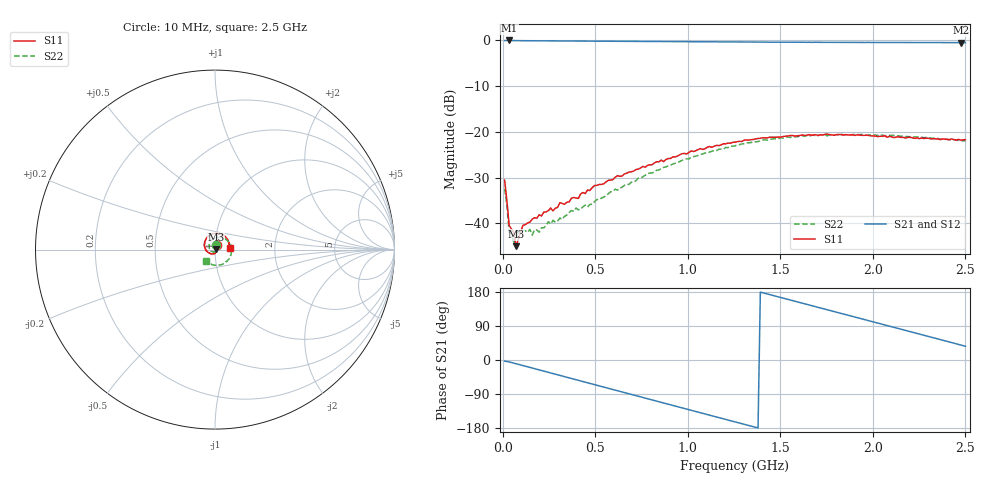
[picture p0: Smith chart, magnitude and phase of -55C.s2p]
!Agilent Technologies,E8364B,MY43040864,A.07.50.48
!Agilent E8364B: A.07.50.48
!Date: Tuesday, September 09, 2025 17:34:12
!Correction: S11(Full 2 Port(1,2))
!S21(Full 2 Port(1,2))
!S12(Full 2 Port(1,2))
!S22(Full 2 Port(1,2))
!S2P File: Measurements: S11, S21, S12, S22:
# Hz S  dB  R 50
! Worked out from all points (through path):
!   201 points, 10 MHz to 2.5 GHz, reference 50 ohm
!   highest |S21| = -0.01 dB at 34.9 MHz (marker M1); lowest = -0.5 dB at 2.475 GHz (marker M2)
!   group delay of S21, straight-line fit = 359 ps
!   lowest |S11| = -45.0 dB at 72.25 MHz (marker M3), VSWR 1.01, Z = 50.6 + j0.134 ohm
!   |S11| at or under -10 dB: start of sweep to end of sweep
!   |S22| runs from -44.5 to -20.5 dB; largest |S21 - S12| = 0.0037
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1e7  -30.53 68.7  -0.03 -2.9  -0.03 -2.9  -32.42 79.3
2.245e7  -35.14 59.1  -0.03 -4.0  -0.04 -4.0  -36.00 70.6
3.49e7  -40.49 52.3  -0.01 -5.2  -0.02 -5.1  -42.06 55.7
4.735e7  -41.23 46.1  -0.03 -6.7  -0.05 -6.7  -42.39 26.8
5.98e7  -42.03 29.8  -0.04 -8.3  -0.07 -8.4  -44.47 37.0
7.225e7  -44.98 13.6  -0.06 -9.9  -0.06 -9.9  -41.28 21.1
1.096e8  -40.39 10.1  -0.07 -14.9  -0.07 -14.8  -41.46 17.6
1.4695e8  -39.70 -18.3  -0.07 -19.6  -0.10 -19.6  -41.30 -20.6
1.594e8  -39.06 -26.3  -0.09 -21.3  -0.09 -21.2  -42.56 -22.2
2.4655e8  -37.21 -54.2  -0.11 -32.6  -0.11 -32.6  -39.62 -57.1
4.333e8  -33.25 -99.3  -0.15 -56.9  -0.16 -56.8  -36.36 -112.4
6.325e8  -29.73 -136.2  -0.20 -82.7  -0.21 -82.8  -32.32 -167.0
8.4415e8  -26.54 -169.7  -0.25 -110.1  -0.25 -110.2  -28.32 147.2
1.06825e9  -23.65 155.7  -0.30 -139.2  -0.30 -139.2  -24.99 107.4
1.255e9  -22.28 129.5  -0.33 -163.3  -0.34 -163.3  -23.08 75.1
1.46665e9  -21.16 102.2  -0.38 169.5  -0.38 169.6  -21.46 41.5
1.6783e9  -20.70 77.8  -0.40 142.4  -0.42 142.3  -20.67 5.9
1.9024e9  -20.77 54.3  -0.43 113.4  -0.45 113.5  -20.51 -29.6
2.08915e9  -20.97 37.3  -0.46 89.4  -0.46 89.4  -20.77 -60.4
2.2759e9  -21.45 22.0  -0.47 65.3  -0.48 65.3  -21.27 -91.4
2.4751e9  -21.81 8.5  -0.49 39.5  -0.49 39.5  -21.86 -125.3
2.5e9  -21.71 6.7  -0.49 36.3  -0.50 36.3  -21.96 -129.6
